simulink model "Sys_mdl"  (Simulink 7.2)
settings: Solver=ode45  StartTime=0.0  StopTime=10.0  RelTol=1e-3
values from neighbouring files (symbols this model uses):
  A = [ -b1/Ma  -K   b1/Mr         0    [Esercitazione04.m]
  B = [-Ma   1   0    [Esercitazione04.m]
  C = [1/Ma  0   0  0]    [Esercitazione04.m]
  g = 9.81    [Esercitazione04.m]
  RispostaForzata = 1    [Esercitazione04.m]
  X0 = [0 0.05 0 0]'    [Esercitazione04.m]

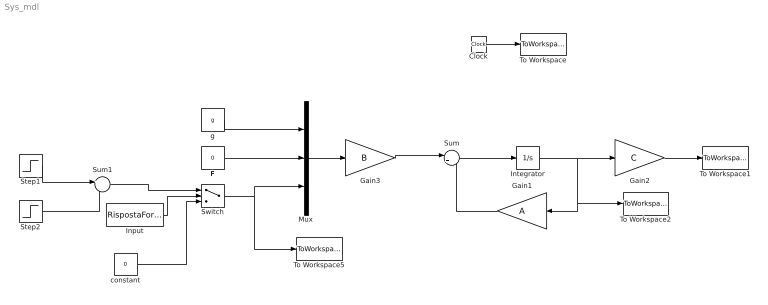
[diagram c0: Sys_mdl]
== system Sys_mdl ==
  Clock : Clock
  F : Constant  Value=0  OutDataType=sfix(16)  OutScaling=2^0
  Gain1 : Gain  Orientation=left  Gain=A  Multiplication=Matrix(K*u)  ParameterDataType=sfix(16)  ParameterScaling=2^0  OutDataType=sfix(16)  OutScaling=2^0
  Gain2 : Gain  Gain=C  Multiplication=Matrix(K*u)  ParameterDataType=sfix(16)  ParameterScaling=2^0  OutDataType=sfix(16)  OutScaling=2^0
  Gain3 : Gain  Gain=B  Multiplication=Matrix(K*u)  ParameterDataType=sfix(16)  ParameterScaling=2^0  OutDataType=sfix(16)  OutScaling=2^0
  Input : Constant  Value=RispostaForzata  OutDataType=sfix(16)  OutScaling=2^0
  Integrator : Integrator  InitialCondition=X0
  Mux : Mux  Inputs=3
  Step1 : Step  Time=5  SampleTime=0
  Step2 : Step  Time=5+0.2  SampleTime=0
  Sum : Sum  Inputs=|++  OutDataType=sfix(16)  OutScaling=2^0
  Sum1 : Sum  Inputs=+-  OutDataType=sfix(16)  OutScaling=2^0
  Switch : Switch  Threshold=0.5  OutDataType=sfix(16)  OutScaling=2^0
  To Workspace : ToWorkspace  VariableName=time  SampleTime=-1  SaveFormat=Array
  To Workspace1 : ToWorkspace  VariableName=y  SampleTime=-1  SaveFormat=Array
  To Workspace2 : ToWorkspace  VariableName=x  SampleTime=-1  SaveFormat=Array
  To Workspace5 : ToWorkspace  VariableName=dXs  SampleTime=-1  SaveFormat=Array
  constant : Constant  Value=0  OutDataType=sfix(16)  OutScaling=2^0
  g : Constant  Value=g  OutDataType=sfix(16)  OutScaling=2^0
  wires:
  Gain3/1 -> Sum/1
  Gain1/1 -> Sum/2
  Sum/1 -> Integrator/1
  Integrator/1 -> Gain2/1, Gain1/1, To Workspace2/1
  Clock/1 -> To Workspace/1
  Gain2/1 -> To Workspace1/1
  Mux/1 -> Gain3/1
  g/1 -> Mux/1
  F/1 -> Mux/2
  Switch/1 -> Mux/3, To Workspace5/1
  Step1/1 -> Sum1/1
  Step2/1 -> Sum1/2
  Sum1/1 -> Switch/1
  Input/1 -> Switch/2
  constant/1 -> Switch/3
